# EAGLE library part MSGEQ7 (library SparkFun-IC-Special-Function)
7-band graphic equalizer This IC is for making a 7 band/channel audio spectrometer. There are two versions of this part. The DIP available on the storefront, and the SO used in product. Datasheet SparkFun Products Storefront component: Graphic Equalizer Display Filter - MSGEQ7 (COM-10468) SparkFun Spectrum Shield (DEV-13116)
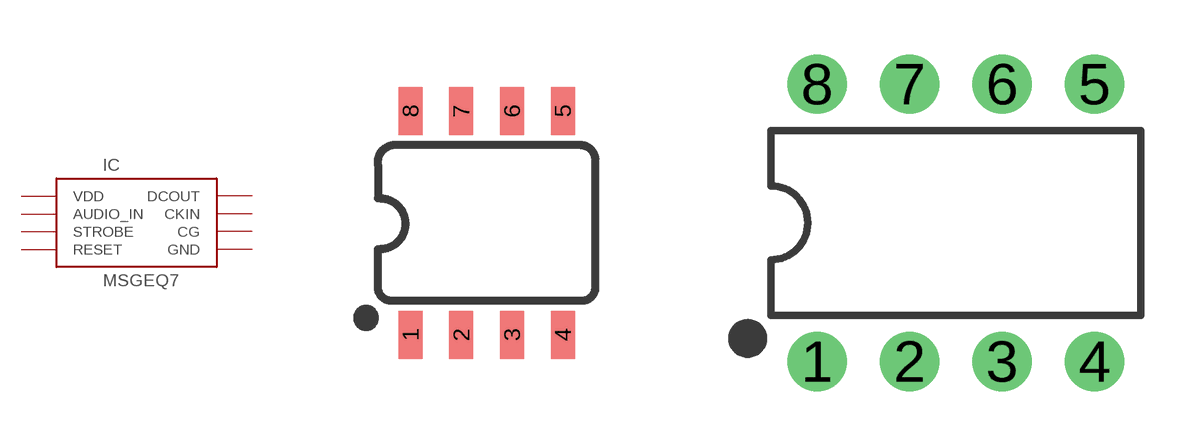
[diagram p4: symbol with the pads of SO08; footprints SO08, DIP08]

Designator prefix IC

## MSGEQ7SOIC (PROD_ID: IC-10141; VALUE: MSGEQ7N)  [SO08]
1  VDD  in
2  GND
3  DCOUT
4  STROBE  in
5  AUDIO_IN  in
6  CG
7  RESET  in
8  CKIN

## MSGEQ7DIL (PROD_ID: IC-12196; VALUE: MSGEQ7P)  [DIP08]
Pads as for SO08

## Footprint SO08 (pad centres in mm)
SOIC, 0.15 inch width
smd 0.6 x 1.2: 1 -1.905,-2.8; 2 -0.635,-2.8; 3 0.635,-2.8; 4 1.905,-2.8; 5 1.905,2.8; 6 0.635,2.8; 7 -0.635,2.8; 8 -1.905,2.8

## Footprint DIP08 (pad centres in mm)
Dual In Line Package
drill 0.813 pad 1.626: 1 -3.81,-3.81; 2 -1.27,-3.81; 3 1.27,-3.81; 4 3.81,-3.81; 5 3.81,3.81; 6 1.27,3.81; 7 -1.27,3.81; 8 -3.81,3.81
